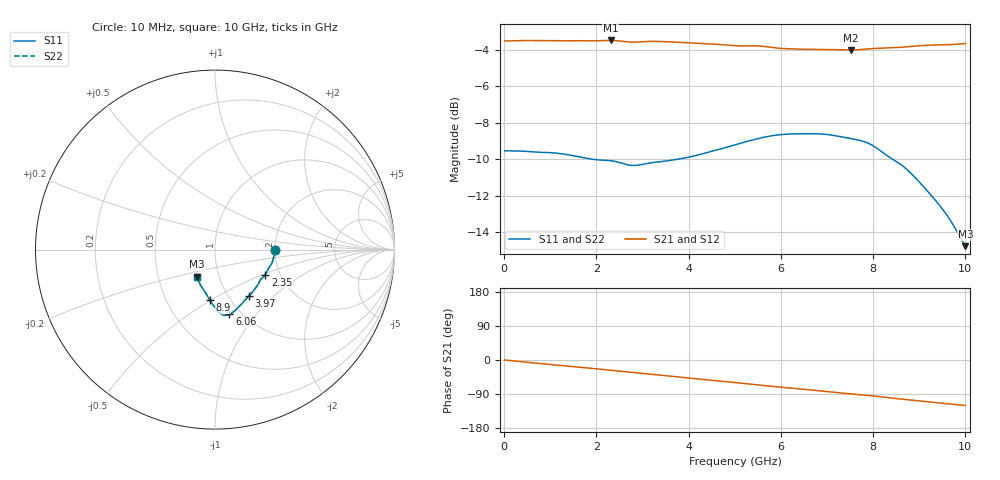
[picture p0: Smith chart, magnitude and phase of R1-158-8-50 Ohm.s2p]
!version-1
!date-10.2020
!Series
#GHZ	S	RI	R	50.0
!FREQ.GHZ	S11RE	S11IM	S21RE	S21IM	S12RE	S12IM	S22RE	S22IM
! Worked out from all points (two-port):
!   500 points, 10 MHz to 10 GHz, reference 50 ohm
!   highest |S21| = -3.49 dB at 2.31 GHz (marker M1); lowest = -4.0 dB at 7.52 GHz (marker M2)
!   |S21| within 3 dB of the highest: start of sweep to end of sweep
!   lowest |S11| = -14.8 dB at 10 GHz (marker M3), VSWR 1.45, Z = 39.1 - j12.2 ohm
!   |S11| at or under -10 dB: 1.907 GHz to 3.764 GHz (1.857 GHz wide, 65.5 % of centre); 8.422 GHz to end of sweep
!   |S22| runs from -14.8 to -8.6 dB; largest |S21 - S12| = 0
!   S11 on the Smith chart (normalised r, x): 10 MHz: 2.00, -0.00; 2.35 GHz: 1.68, -0.52; 3.97 GHz: 1.24, -0.71; 6.06 GHz: 0.88, -0.74; 8.9 GHz: 0.81, -0.49; 10 GHz: 0.78, -0.24
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0.01  0.3333 -0.000619  0.6666 -0.0014  0.6666 -0.0014  0.3333 -0.000619
0.751  0.3282 -0.0381  0.6602 -0.1035  0.6602 -0.1035  0.3282 -0.0381
1.13  0.323 -0.0602  0.6498 -0.1524  0.6498 -0.1524  0.323 -0.0602
1.69  0.3063 -0.0919  0.63 -0.2212  0.63 -0.2212  0.3063 -0.0919
2.31  0.2818 -0.1366  0.5961 -0.3034  0.5961 -0.3034  0.2818 -0.1366
2.35  0.2798 -0.1397  0.5934 -0.3084  0.5934 -0.3084  0.2798 -0.1397
2.79  0.2531 -0.1681  0.5548 -0.3606  0.5548 -0.3606  0.2531 -0.1681
3.35  0.2286 -0.2106  0.5134 -0.4223  0.5134 -0.4223  0.2286 -0.2106
3.97  0.1889 -0.2579  0.4479 -0.4836  0.4479 -0.4836  0.1889 -0.2579
4.53  0.1568 -0.2939  0.384 -0.5293  0.384 -0.5293  0.1568 -0.2939
5.02  0.1301 -0.3212  0.3271 -0.5581  0.3271 -0.5581  0.1301 -0.3212
5.54  0.1044 -0.3455  0.2608 -0.5908  0.2608 -0.5908  0.1044 -0.3455
6.06  0.0805 -0.3609  0.1918 -0.6058  0.1918 -0.6058  0.0805 -0.3609
6.68  0.06 -0.3665  0.1162 -0.6215  0.1162 -0.6215  0.06 -0.3665
7.26  0.0426 -0.3626  0.0378 -0.6298  0.0378 -0.6298  0.0426 -0.3626
7.52  0.0382 -0.3582  0.00728 -0.6298  0.00728 -0.6298  0.0382 -0.3582
7.92  0.0182 -0.3481  -0.0406 -0.6334  -0.0406 -0.6334  0.0182 -0.3481
8.34  0.000612 -0.321  -0.1077 -0.6291  -0.1077 -0.6291  0.000612 -0.321
8.64  -0.0151 -0.3026  -0.1487 -0.6237  -0.1487 -0.6237  -0.0151 -0.3026
8.9  -0.0282 -0.2811  -0.1818 -0.6195  -0.1818 -0.6195  -0.0282 -0.2811
9.54  -0.0687 -0.2169  -0.2703 -0.5919  -0.2703 -0.5919  -0.0687 -0.2169
10  -0.1021 -0.1514  -0.327 -0.5689  -0.327 -0.5689  -0.1021 -0.1514
